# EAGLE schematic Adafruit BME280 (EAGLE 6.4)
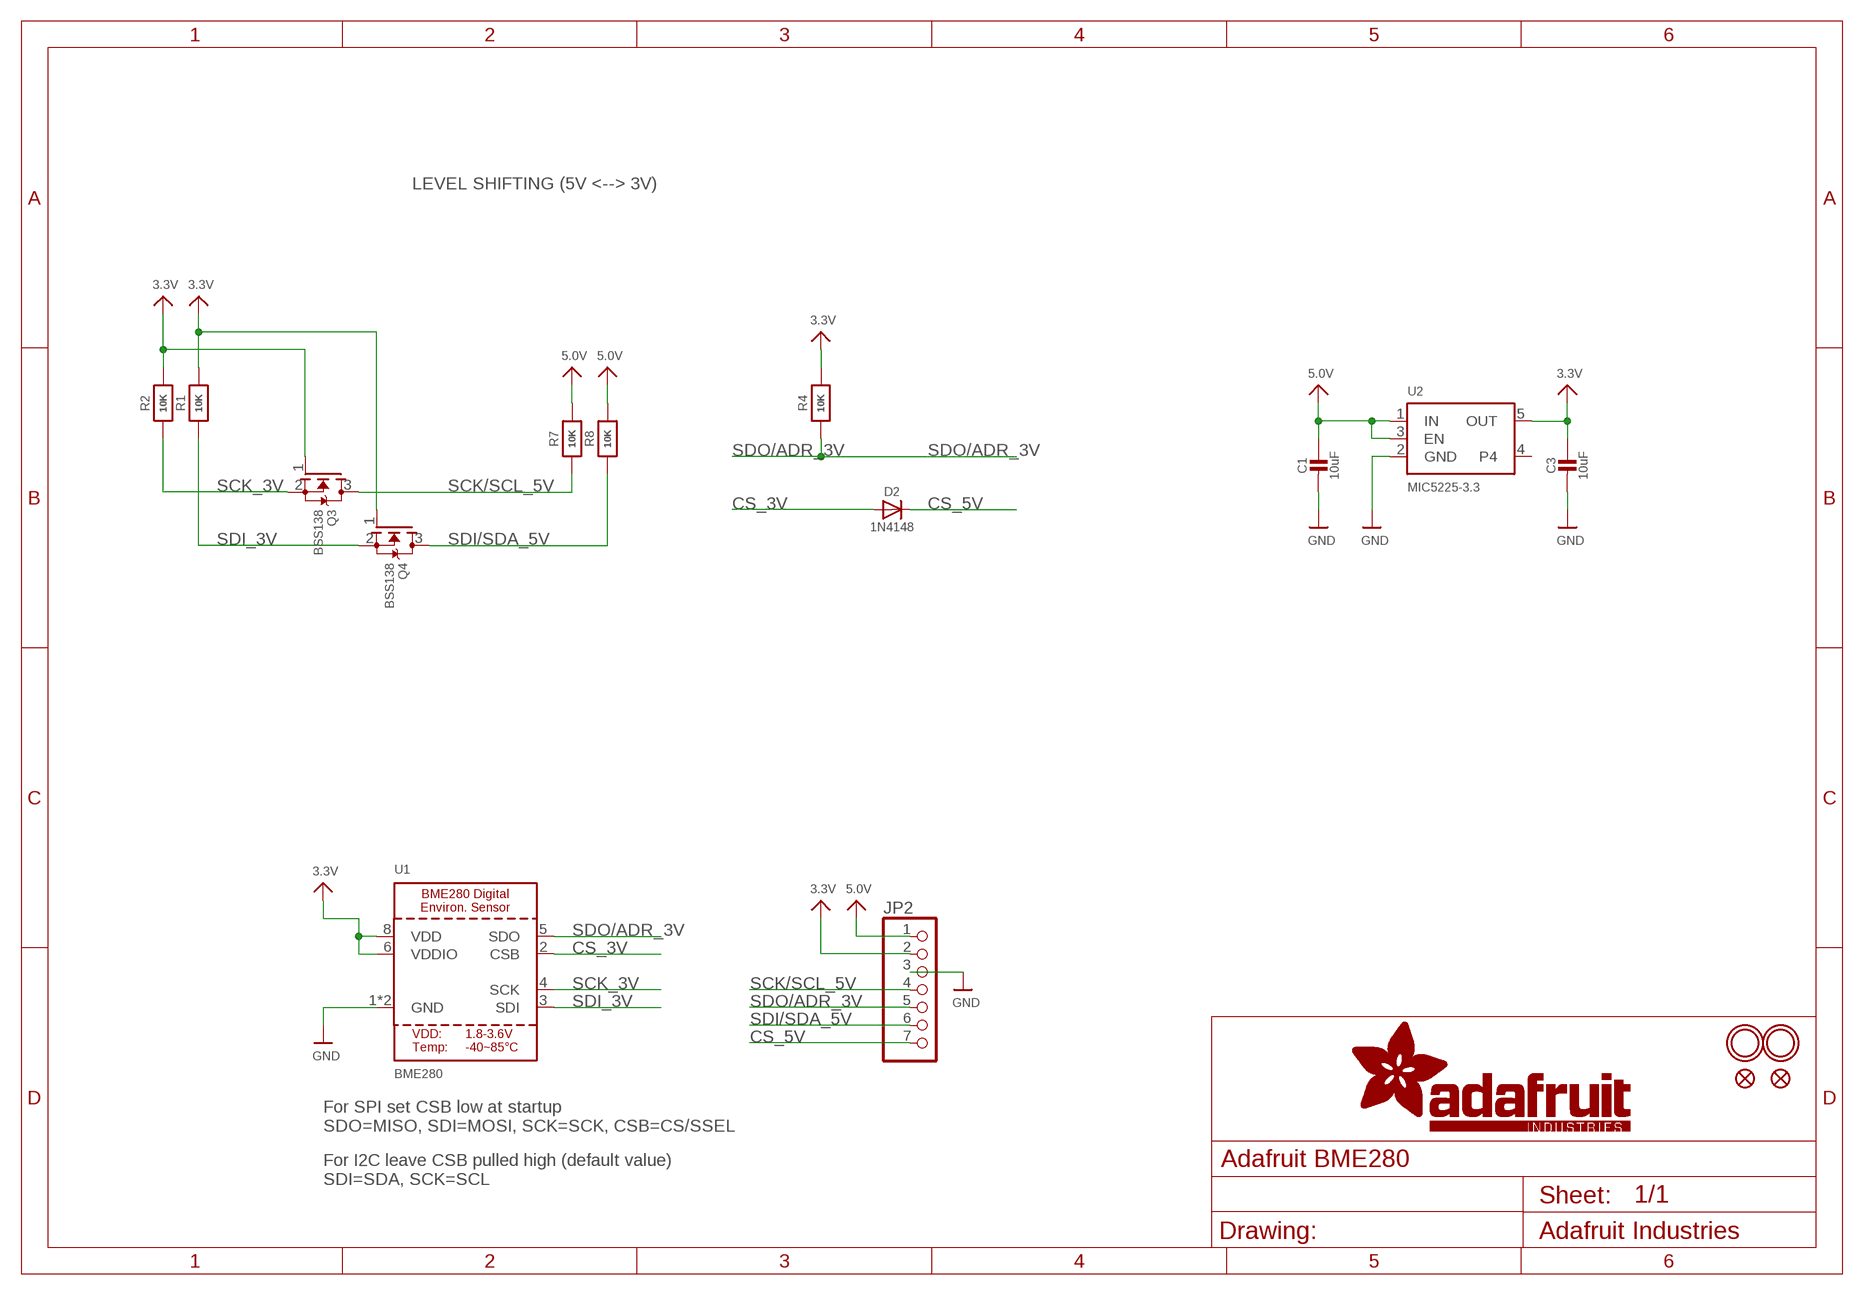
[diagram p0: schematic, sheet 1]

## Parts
C1  10uF  CAP_CERAMIC0805-NOOUTLINE  [0805-NO]
C3  10uF  CAP_CERAMIC0805-NOOUTLINE  [0805-NO]
D2  1N4148  DIODESOD-323  [SOD-323]
JP2  HEADER-1X770MIL  [1X07_ROUND_70]
Q3  BSS138  MOSFET-NWIDE  [SOT23-WIDE]
Q4  BSS138  MOSFET-NWIDE  [SOT23-WIDE]
R1  10K  RESISTOR0805_NOOUTLINE  [0805-NO]
R2  10K  RESISTOR0805_NOOUTLINE  [0805-NO]
R4  10K  RESISTOR_0805MP  [_0805MP]
R7  10K  RESISTOR0805_NOOUTLINE  [0805-NO]
R8  10K  RESISTOR0805_NOOUTLINE  [0805-NO]
U1  BME280  [BME280]
U2  MIC5225-3.3  VREG_SOT23-5  [SOT23-5]
U$5  FIDUCIAL""  [FIDUCIAL_1MM]
U$7  MOUNTINGHOLE2.0  [MOUNTINGHOLE_2.0_PLATED]
U$8  MOUNTINGHOLE2.0  [MOUNTINGHOLE_2.0_PLATED]
U$15  FIDUCIAL""  [FIDUCIAL_1MM]

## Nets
3.3V: C3.1 JP2.2 Q3.1(G) Q4.1(G) R1.2 R2.2 R4.2 U1.6(VDDIO) U1.8(VDD) U2.5(OUT)
5.0V: C1.1 JP2.1 R7.2 R8.2 U2.1(IN) U2.3(EN)
CS_3V: D2.A U1.2(CSB)
CS_5V: D2.C JP2.7
GND: C1.2 C3.2 JP2.3 U1.1(GND) U1.7(GND) U2.2(GND)
SCK/SCL_5V: JP2.4 Q3.3(D) R7.1
SCK_3V: Q3.2(S) R2.1 U1.4(SCK)
SDI/SDA_5V: JP2.6 Q4.3(D) R8.1
SDI_3V: Q4.2(S) R1.1 U1.3(SDI)
SDO/ADR_3V: JP2.5 R4.1 U1.5(SDO)
Unconnected: U2.4

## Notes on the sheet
- LEVEL SHIFTING (5V <--> 3V)
- For SPI set CSB low at startup
  SDO=MISO, SDI=MOSI, SCK=SCK, CSB=CS/SSEL
- For I2C leave CSB pulled high (default value)
  SDI=SDA, SCK=SCL

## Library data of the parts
C1 C3 = microbuilder:CAP_CERAMIC: Ceramic Capacitors
D2 = microbuilder:DIODE: Diode
JP2 = microbuilder:HEADER-1X7: PIN HEADER
Q3 Q4 = microbuilder:MOSFET-N: N-Channel Mosfet LEGEND VDS: Voltage Drain-Source ID: Drain Current RDS(ON): Drain-Source On-State Resistance VGS(TH): Gate-Source Threshold Voltage CISS: Drain-Source Input Capacitance SOT-23 Name VDS ID RDS(ON) VGS(TH) CISS Order Number 2N7002E 60V 260mA 2.5 Ohm 2.5V @ 250uA 26.7pF @ 25V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
R1 R2 R4 R7 R8 = microbuilder:RESISTOR: Resistors
U1 = microbuilder:BME280: BME280 - Environmental Sensor (I2C + SPI)
U2 = microbuilder:VREG_SOT23-5: SOT23-5 Fixed Voltage Regulators Part Current Out V Out V In V Dropout θJA (°C/W) TJ (°C) Digikey Part No. ADP121 150mA 3.3V 3.4-5.5V 0.09V @ 150mA -- -- ADP121-AUJZ33R7CT-ND ADP121 150mA 3.0V 3.1-5.5V 0.09V @ 150mA -- -- ADP121-AUJZ30R7CT-ND ADP122 300mA 3.3V 3.4-5.5V 0.085V @ 300mA -- --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
U$5 U$15 = microbuilder:FIDUCIAL: Fiducial Alignment Points; BOM: EXCLUDE
U$7 U$8 = microbuilder:MOUNTINGHOLE: Mounting Hole; BOM: EXCLUDE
